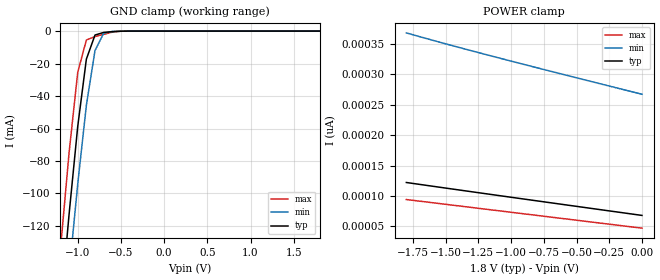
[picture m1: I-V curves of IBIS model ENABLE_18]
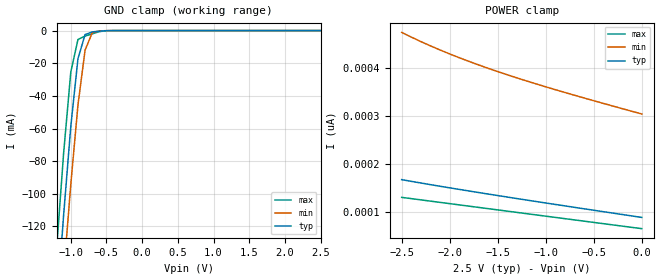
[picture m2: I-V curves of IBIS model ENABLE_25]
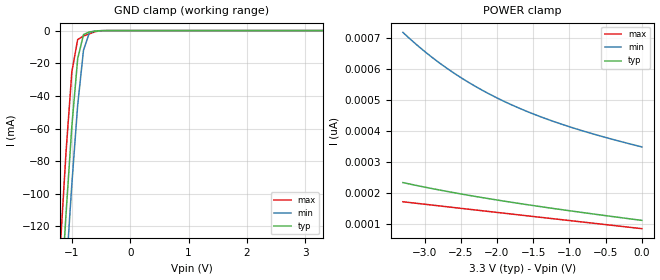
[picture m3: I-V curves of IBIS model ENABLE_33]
|   @@@@@@@   @@@@@@@   @@@@@@@   @@@@@@@   @@@@@@@   @@@@@@   @@
|   @@@@@@@@@   @@@@@@@@@   @@@@@@@@@   @@@@@@@@@   @@@@@@@@@ @@@@@@@@  @
|   @@@   @@@ @@@   @@@ @@@   @@@   @@@ @@@   @@@@   @@@  @
|   @@   @@ @@   @@ @@@@@@@@@@@ @@@@@@@@@@@ @@   @@   @@ @@
|   @@@   @@@ @@   @@   @@@ @@@   @@   @@   @@ @@
|   @@@@@@@@@  @@   @@  @@@@@@@@@   @@@@@@@@@  @@   @@   @@ @@
|   @@@@@@@   @@   @@   @@@@@@@   @@@@@@@   @@   @@   @@ @@
|   IBIS Model of NL5X4002
|   2-Bit 24 Mbps Configurable Dual-Supply Autosense Level Translator
|   Package Type:
|   SOIC-8 NB, CASE 751
|   Micro8, CASE 846A
|   UDFN8, CASE 517AJ, CASE 517BZ
|   UQFN8, CASE 523AS
|   This device can be powered at following Vccs:
|   1.8 volt
|   2.5 volt
|   3.3 volt
|   5.0 volt
|   To operate at each Vcc, select the appropriate model in [Model Selector]
[IBIS Ver]   3.2
[Comment Char]   |_char
[File name]   nl5x4002_85c_sa_r0.ibs
[File Rev]   0.0
[Date]   June 25, 2025
[Source]
SPICE to IBIS translation
[Notes]
No Power clamp data specified for there is no power clamp diode.
[Disclaimer]
- onsemi Corporation hereby grants
the user of this IBIS model a license to use this IBIS
model under the following terms. This license in nonexclusive
and nontransferable. Before using this IBIS model.
After reading the terms and conditions of this license,
the user either must accept these terms,
or the IBIS model should be returned to onsemi within 30 days.
- The user is hereby granted a license to use the IBIS model.
This shall not be construed as a right to sell,
or otherwise profit either by leasing or renting this software.
- The user may modify the IBIS model to suit his specific
applications but rights to derivative works and such
modifications shall belong to onsemi.
- This IBIS model is provided on an "as is" basis.
onsemi makes absolutely no warranty with respect
to the information contained herein.
By use of this IBIS model, the user assumes full risk as to the
quality and suitablility of the model to his particular use,
and by using this model assumes the entire risk.
Under all circumstances the user shall not hold
onsemi liable in any way for the results obtained.
onsemi reserves the right to make to improve
the model for reliability, function, or design.
onsemi does not convey any license under patent
rights or any other intellectual property rights,
including those of third parties.
- onsemi is not obligated to provide maintenance
or support for the licensed IBIS model.
- Cont onsemi at ATTN:LOGIC APPLICATIONS/IBIS MODEL.
5005 E. McDowell Road, Phoenix AZ 85008
[Copyright]
   (c) 2025 onsemi Corp.
[Component]   NL5X4002DR2G
|  SOIC-8 NB
|   CASE 751
Si_location Die
Timing_location Die
[Manufacturer]   onsemi
|   Data Sheet: NL5X4002-D, Rev. 0,  June, 2025
[Package]
R_pkg   0.0388   0.0343   0.0438
L_pkg   5.0121nH   4.1117nH   6.34108nH
C_pkg   0.7179pF   0.532pF   0.8677pF
[Pin] signal_name   model_name   R_pin   L_pin   C_pin
1   VCCA   POWER   0.0438   6.3361nH   0.8661pF
2   A1   IO   0.0438   5.5422nH   0.8677pF
3   A2   IO   0.0352   4.7156nH   0.7335pF
4   GND   GND   0.0358   4.3786nH   0.5920pF
5   EN   ENABLE   0.0362   4.1319nH   0.5345pF
6   B2   IO   0.0352   4.1126nH   0.5320pF
7   B1   IO   0.0346   4.2858nH   0.5830pF
8   VCCB   POWER   0.0343   4.6345nH   0.7277pF
[Component]   NL5X4002DR2G-Q
|  SOIC-8 NB
|   CASE 751
Si_location Die
Timing_location Die
[Manufacturer]   onsemi
|   Data Sheet: NL5X4002-D, Rev. 0,  June, 2025
[Package]
R_pkg   0.0388   0.0343   0.0438
L_pkg   5.0121nH   4.1117nH   6.34108nH
C_pkg   0.7179pF   0.532pF   0.8677pF
[Pin] signal_name   model_name   R_pin   L_pin   C_pin
1   VCCA   POWER   0.0438   6.3361nH   0.8661pF
2   A1   IO   0.0438   5.5422nH   0.8677pF
3   A2   IO   0.0352   4.7156nH   0.7335pF
4   GND   GND   0.0358   4.3786nH   0.5920pF
5   EN   ENABLE   0.0362   4.1319nH   0.5345pF
6   B2   IO   0.0352   4.1126nH   0.5320pF
7   B1   IO   0.0346   4.2858nH   0.5830pF
8   VCCB   POWER   0.0343   4.6345nH   0.7277pF
[Component]   NL5X4002MU3TAG
|   UDFN_8
| CASE 517BZ
Si_location Die
Timing_location Die
[Manufacturer]   onsemi
|   Data Sheet: NL5X4002-D, Rev. 0,  June, 2025
[Package]
R_pkg   0.0406   0.0262   0.0540
L_pkg   0.3578nH   0.296nH   0.4397nH
C_pkg   0.0584pF   0.0517pF   0.06777pF
[Pin] signal_name   model_name   R_pin   L_pin   C_pin
1   VCCA   POWER   0.0262   0.3020nH   0.0654pF
2   A1   IO   0.0479   0.3748nH   0.0527pF
3   A2   IO   0.0479   0.3822nH   0.0557pF
4   GND   GND   0.0273   0.3218nH   0.0678pF
5   EN   ENABLE   0.0540   0.4397nH   0.0528pF
6   B2   IO   0.0479   0.3765nH   0.0517pF
7   B1   IO   0.0472   0.3694nH   0.0548pF
8   VCCB   POWER   0.0262   0.2960nH   0.0659pF
[Component]   NL5X4002MU3TCG
|   UDFN_8
| CASE 517BZ
Si_location Die
Timing_location Die
[Manufacturer]   onsemi
|   Data Sheet: NL5X4002-D, Rev. 0,  June, 2025
[Package]
R_pkg   0.0406   0.0262   0.0540
L_pkg   0.3578nH   0.296nH   0.4397nH
C_pkg   0.0584pF   0.0517pF   0.06777pF
[Pin] signal_name   model_name   R_pin   L_pin   C_pin
1   VCCA   POWER   0.0262   0.3020nH   0.0654pF
2   A1   IO   0.0479   0.3748nH   0.0527pF
3   A2   IO   0.0479   0.3822nH   0.0557pF
4   GND   GND   0.0273   0.3218nH   0.0678pF
5   EN   ENABLE   0.0540   0.4397nH   0.0528pF
6   B2   IO   0.0479   0.3765nH   0.0517pF
7   B1   IO   0.0472   0.3694nH   0.0548pF
8   VCCB   POWER   0.0262   0.2960nH   0.0659pF
[Component]   NL5X4002MUTAG
|   UDFN_8
| CASE 517AJ
Si_location Die
Timing_location Die
[Manufacturer]   onsemi
|   Data Sheet: NL5X4002-D, Rev. 0,  June, 2025
[Package]
R_pkg   0.0451   0.0011   0.0571
L_pkg   0.3714nH   0.01454nH   0.4787nH
C_pkg   0.1048pF   0.07664pF   0.1133pF
[Pin] signal_name   model_name   R_pin   L_pin   C_pin
1   VCCA   POWER   0.0486   0.3921nH  0.1052pF
2   A1   IO   0.0469   0.3815nH  0.1078pF
3   A2   IO   0.0570   0.4787nH  0.1129pF
4   GND   GND   0.0544   0.4523nH  0.1100pF
5   EN   ENABLE   0.0011   0.0145nH  0.0766pF
6   B2   IO   0.0571   0.4787nH  0.1133pF
7   B1   IO   0.0470   0.3814nH  0.1077pF
8   VCCB   POWER   0.0486   0.3922nH  0.1052pF
[Component]   NL5X4002MUTAG-Q
|   UDFN_8
| CASE 517AJ
Si_location Die
Timing_location Die
[Manufacturer]   onsemi
|   Data Sheet: NL5X4002-D, Rev. 0,  June, 2025
[Package]
R_pkg   0.0451   0.0011   0.0571
L_pkg   0.3714nH   0.01454nH   0.4787nH
C_pkg   0.1048pF   0.07664pF   0.1133pF
[Pin] signal_name   model_name   R_pin   L_pin   C_pin
1   VCCA   POWER   0.0486   0.3921nH  0.1052pF
2   A1   IO   0.0469   0.3815nH  0.1078pF
3   A2   IO   0.0570   0.4787nH  0.1129pF
4   GND   GND   0.0544   0.4523nH  0.1100pF
5   EN   ENABLE   0.0011   0.0145nH  0.0766pF
6   B2   IO   0.0571   0.4787nH  0.1133pF
7   B1   IO   0.0470   0.3814nH  0.1077pF
8   VCCB   POWER   0.0486   0.3922nH  0.1052pF
[Component]   NL5X4002DMR2G
|   Micro8
| CASE 846A-02
Si_location Die
Timing_location Die
[Manufacturer]   onsemi
|   Data Sheet: NL5X4002-D, Rev. 0,  June, 2025
[Package]
R_pkg   0.1829   0.0061   0.2446
L_pkg   2.8385nH   1.565nH   3.89485nH
C_pkg   0.4567pF   0.38386pF   0.53234pF
[Pin] signal_name   model_name   R_pin   L_pin   C_pin
1   VCCA   POWER   0.1862   2.8664nH   0.4560pF
2   A1   IO   0.2446   3.8949nH   0.5323pF
3   A2   IO   0.2357   3.2912nH   0.4714pF
4   GND   GND   0.1867   2.8664nH   0.4559pF
5   EN   ENABLE   0.1866   1.5684nH   0.3839pF
6   B2   IO   0.2341   3.8112nH   0.5277pF
7   B1   IO   0.0061   1.5650nH   0.3853pF
8   VCCB   POWER   0.1830   2.8445nH   0.4412pF
[Component]   NL5X4002DMR2G-Q
|   Micro8
| CASE 846A-02
Si_location Die
Timing_location Die
[Manufacturer]   onsemi
|   Data Sheet: NL5X4002-D, Rev. 0,  June, 2025
[Package]
R_pkg   0.1829   0.0061   0.2446
L_pkg   2.8385nH   1.565nH   3.89485nH
C_pkg   0.4567pF   0.38386pF   0.53234pF
[Pin] signal_name   model_name   R_pin   L_pin   C_pin
1   VCCA   POWER   0.1862   2.8664nH   0.4560pF
2   A1   IO   0.2446   3.8949nH   0.5323pF
3   A2   IO   0.2357   3.2912nH   0.4714pF
4   GND   GND   0.1867   2.8664nH   0.4559pF
5   EN   ENABLE   0.1866   1.5684nH   0.3839pF
6   B2   IO   0.2341   3.8112nH   0.5277pF
7   B1   IO   0.0061   1.5650nH   0.3853pF
8   VCCB   POWER   0.1830   2.8445nH   0.4412pF
[Component]   NL5X4002MQ2TCG
|   UQFN-8
| CASE 523AS
Si_location Die
Timing_location Die
[Manufacturer]   onsemi
|   Data Sheet: NL5X4002-D, Rev. 0,  June, 2025
[Package]
R_pkg   0.0427   0.0377   0.0476
L_pkg   0.483n   0.412n   0.526n
C_pkg   0.068p   0.066p   0.076p
[Pin] signal_name   model_name   R_pin   L_pin   C_pin
1   VCCA   POWER   45.8m   0.499n   0.076p
2   A1   IO   42.7m   0.483n   0.068p
3   A2   IO   41.3m   0.464n   0.067p
4   GND   GND   43.9m   0.479n   0.066p
5   EN   ENABLE   47.6m   0.526n   0.067p
6   B2   IO   43.8m   0.493n   0.070p
7   B1   IO   41.4m   0.459n   0.068p
8   VCCB   POWER   37.7m   0.412n   0.067p
[Model Selector]   IO
IO_18   1.8V Vcc
IO_25   2.5V Vcc
IO_33   3.3V Vcc
IO_50   5.0V Vcc
[Model Selector]   ENABLE
ENABLE_18   1.8V Vcc
ENABLE_25   2.5V Vcc
ENABLE_33   3.3V Vcc
ENABLE_50   5.0V Vcc
| Models and submodels in the file (8): ENABLE_18 (Input), ENABLE_25 (Input), ENABLE_33 (Input), ENABLE_50 (Input), IO_18 (I/O_open_drain), IO_25 (I/O_open_drain), IO_33 (I/O_open_drain), IO_50 (I/O_open_drain)
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[Model]   ENABLE_18
Model_type Input
Vinh=1.26
Vinl=0.54
C_comp   4.0p   NA   NA
[Model Spec]
Vinh   1.26   1.155   1.365
Vinl   0.54   0.495   0.585
[Temperature Range] 25   85   -40
[Voltage Range]   1.8   1.65   1.95
[Pullup Reference]  1.8   1.65   1.95
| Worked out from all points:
|   GND clamp passes 1 mA (typ) near -0.71 V on its own axis
[GND Clamp]
-1.8V     -552.9mA   -576.3mA   -528.9mA
-1.2V     -171.7mA   -206.9mA   -134.3mA
-1.1V     -112.8mA   -149mA     -74.83mA
-1V       -58.71mA   -94.21mA   -25.39mA
-900mV    -17.28mA   -45.7mA    -5.488mA
-800mV    -2.447mA   -11.99mA   -3.347mA
-700mV    -836.3uA   -1.356mA   -2.02mA
-600mV    -357.3uA   -195.6uA   -652.3uA
-500mV    -83.24uA   -50.15uA   -83.18uA
1.8V      68.09pA    267pA      47.17pA
[POWER Clamp]
-1.8V     122.1pA    367.6pA    94.15pA
-1.5V     113pA      349.7pA    86.32pA
-1.1V     100.9pA    326.9pA    75.88pA
0V        68.09pA    267pA      47.17pA
[Model]   ENABLE_25
Model_type Input
Vinh=1.75
Vinl=0.75
C_comp   4.0p   NA   NA
[Model Spec]
Vinh   1.75   1.61   1.89
Vinl   0.75   0.69   0.81
[Temperature Range] 25   85   -40
[Voltage Range]   2.5   2.3   2.7
[Pullup Reference]  2.5   2.3   2.7
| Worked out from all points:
|   GND clamp passes 1 mA (typ) near -0.71 V on its own axis
[GND Clamp]
-2.5V     -1.013A    -1.022A    -1.005A
-1.2V     -171.7mA   -206.9mA   -134.3mA
-1.1V     -112.8mA   -149mA     -74.83mA
-1V       -58.71mA   -94.21mA   -25.39mA
-900mV    -17.28mA   -45.7mA    -5.488mA
-800mV    -2.447mA   -11.99mA   -3.347mA
-700mV    -836.3uA   -1.356mA   -2.02mA
-600mV    -357.3uA   -195.6uA   -652.3uA
-400mV    -8.492uA   -9.966uA   -5.196uA
2.5V      88.92pA    304.8pA    65.44pA
[POWER Clamp]
-2.5V     167.7pA    475.1pA    130.8pA
-2.3V     160.8pA    456pA      125.5pA
-2V       150.7pA    430.2pA    117.7pA
-1.8V     144.1pA    414.7pA    112.4pA
-1.5V     134.6pA    393.4pA    104.6pA
-1.2V     125.2pA    373.8pA    96.76pA
-900mV    116pA      355.6pA    88.93pA
0V        88.92pA    304.8pA    65.44pA
[Model]   ENABLE_33
Model_type Input
Vinh=2.31
Vinl=0.99
C_comp   4.0p   NA   NA
[Model Spec]
Vinh   2.31   2.10   2.52
Vinl   0.99   0.90   1.08
[Temperature Range] 25   85   -40
[Voltage Range]   3.3   3.0   3.6
[Pullup Reference]  3.3   3.0   3.6
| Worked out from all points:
|   GND clamp passes 1 mA (typ) near -0.71 V on its own axis
[GND Clamp]
-3.3V     -1.544A    -1.536A    -1.554A
-1.2V     -171.7mA   -206.9mA   -134.3mA
-1.1V     -112.8mA   -149mA     -74.83mA
-1V       -58.71mA   -94.21mA   -25.39mA
-900mV    -17.28mA   -45.7mA    -5.488mA
-800mV    -2.447mA   -11.99mA   -3.347mA
-700mV    -836.3uA   -1.356mA   -2.02mA
-600mV    -357.3uA   -195.6uA   -652.3uA
-400mV    -8.492uA   -9.966uA   -5.196uA
3.3V      113pA      349.7pA    86.32pA
[POWER Clamp]
-3.3V     234.7pA    718.7pA    173pA
-3V       220.2pA    657.3pA    165pA
-2.8V     211.1pA    621.1pA    159.7pA
-2.6V     202.4pA    588.3pA    154.5pA
-2.3V     190.2pA    544.9pA    146.5pA
-2.1V     182.4pA    519.3pA    141.3pA
-1.9V     174.9pA    496.2pA    136pA
-1.5V     160.8pA    456pA      125.5pA
-1.1V     147.4pA    422.3pA    115.1pA
-600mV    131.4pA    386.7pA    102pA
0V        113pA      349.7pA    86.32pA
